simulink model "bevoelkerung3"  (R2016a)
settings: Solver=ode45  StartTime=0.0  StopTime=300  MaxStep=5  RelTol=1e-3
undefined symbols (not defined in the file or in its folder): k, m0

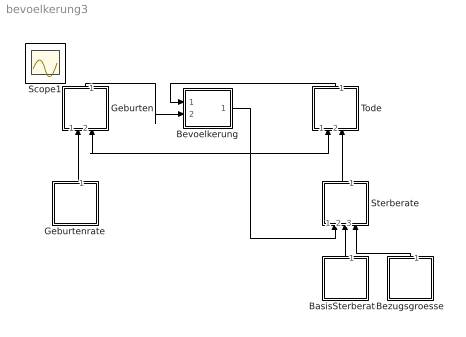
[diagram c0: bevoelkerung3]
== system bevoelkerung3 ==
  BasisSterberate : Subsystem
  Bevoelkerung : Subsystem
  Bezugsgroesse : Subsystem
  Geburten : Subsystem
  Geburtenrate : Subsystem
  Sterberate : Subsystem
  Tode : Subsystem
  Scope1 : Scope
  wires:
  Geburtenrate/1(Out1) -> Geburten/1(In1)
  Geburten/1(Out1) -> Bevoelkerung/2(In2)
  Tode/1(Out1) -> Bevoelkerung/1(In1)
  Sterberate/1(Out1) -> Tode/2(In2)
  BasisSterberate/1(Out1) -> Sterberate/2(In2)
  Bezugsgroesse/1(Out1) -> Sterberate/3(In3)
  Bevoelkerung/1(Out1) -> Sterberate/1(In1), Tode/1(In1), Geburten/2(In2)

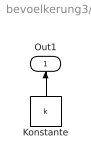
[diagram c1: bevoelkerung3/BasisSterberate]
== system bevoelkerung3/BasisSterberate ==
  Konstante : Constant  Value=k
  Out1 : Outport
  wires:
  Konstante/1 -> Out1/1

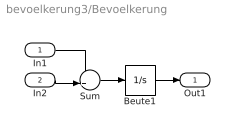
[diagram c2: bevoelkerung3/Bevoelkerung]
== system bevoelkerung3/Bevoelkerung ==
  In1 : Inport
  In2 : Inport  Port=2
  Beute1 : Integrator  InitialCondition=m0
  Sum : Sum  Inputs=-+|
  Out1 : Outport
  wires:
  Sum/1 -> Beute1/1
  In1/1 -> Sum/1
  Beute1/1 -> Out1/1
  In2/1 -> Sum/2

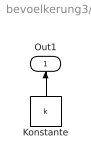
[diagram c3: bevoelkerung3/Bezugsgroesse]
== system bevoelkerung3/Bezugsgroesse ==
  Konstante : Constant  Value=k
  Out1 : Outport
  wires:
  Konstante/1 -> Out1/1

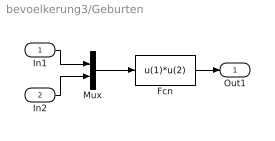
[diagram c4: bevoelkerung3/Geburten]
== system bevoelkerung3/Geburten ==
  In1 : Inport
  In2 : Inport  Port=2
  Fcn : Fcn  Expr=u(1)*u(2)
  Mux : Mux  Inputs=2
  Out1 : Outport
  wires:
  Fcn/1 -> Out1/1
  Mux/1 -> Fcn/1
  In1/1 -> Mux/1
  In2/1 -> Mux/2

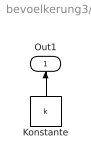
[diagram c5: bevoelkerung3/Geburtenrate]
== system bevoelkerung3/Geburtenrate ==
  Konstante : Constant  Value=k
  Out1 : Outport
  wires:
  Konstante/1 -> Out1/1

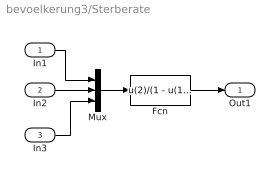
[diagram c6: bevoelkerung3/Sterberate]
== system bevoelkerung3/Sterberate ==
  In1 : Inport
  In2 : Inport  Port=2
  In3 : Inport  Port=3
  Fcn : Fcn  Expr=u(2)/(1 - u(1)/u(3))
  Mux : Mux  Inputs=3
  Out1 : Outport
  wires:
  Fcn/1 -> Out1/1
  Mux/1 -> Fcn/1
  In1/1 -> Mux/1
  In2/1 -> Mux/2
  In3/1 -> Mux/3

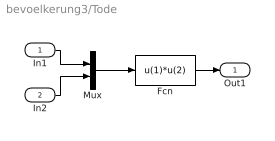
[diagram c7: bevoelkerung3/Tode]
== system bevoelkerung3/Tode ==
  In1 : Inport
  In2 : Inport  Port=2
  Fcn : Fcn  Expr=u(1)*u(2)
  Mux : Mux  Inputs=2
  Out1 : Outport
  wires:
  Fcn/1 -> Out1/1
  Mux/1 -> Fcn/1
  In1/1 -> Mux/1
  In2/1 -> Mux/2
